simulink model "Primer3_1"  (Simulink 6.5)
settings: Solver=ode23t  SolverMode=SingleTasking  StartTime=0.0  StopTime=0.1  RelTol=1e-3  AbsTol=1e-6
undefined symbols (not defined in the file or in its folder): blocks, Continuous, powergui, ZData
libraries: powerlib x17

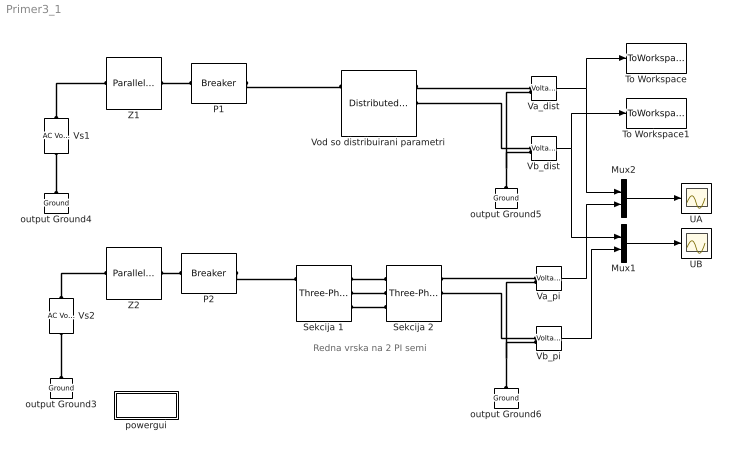
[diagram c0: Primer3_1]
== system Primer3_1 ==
  note: Redna vrska na 2 PI semi
  Mux1 : Mux  Inputs=2
  Mux2 : Mux  Inputs=2
  P1 : powerlib/Elements/Breaker  DialogController=PMDialogs.PMDefaultMaskDlg  SystemSampleTime=-1  BreakerResistance=0.01  InitialState=0  SnubberResistance=inf  SnubberCapacitance=inf  SwitchingTimes="[ 0.25/50  4/50 ]"  External=off  Measurements=None  MoreParameters=off  NoBreakLoop=off
  P2 : powerlib/Elements/Breaker  DialogController=PMDialogs.PMDefaultMaskDlg  SystemSampleTime=-1  BreakerResistance=0.01  InitialState=0  SnubberResistance=inf  SnubberCapacitance=inf  SwitchingTimes="[ 0.25/50  4/50 ]"  External=off  Measurements=None  MoreParameters=off  NoBreakLoop=off
  Sekcija 1 : powerlib/Elements/Three-Phase PI Section Line  DialogController=PMDialogs.PMDefaultMaskDlg  PhysicalDomain=powersysdomain  SubClassName=unknown  LeftPortType=p1  RightPortType=p1  LConnTagsString=a|b|c  RConnTagsString=A|B|C  Frequency=50  Resistances=[0.029983 0.29405]  Inductances=[0.0010055 0.0025377]  Capacitances=[1.1784e-008 8.6541e-009]  Length=113.5/2
  Sekcija 2 : powerlib/Elements/Three-Phase PI Section Line  DialogController=PMDialogs.PMDefaultMaskDlg  PhysicalDomain=powersysdomain  SubClassName=unknown  LeftPortType=p1  RightPortType=p1  LConnTagsString=a|b|c  RConnTagsString=A|B|C  Frequency=50  Resistances=[0.029983 0.29405]  Inductances=[0.0010055 0.0025377]  Capacitances=[1.1784e-008 8.6541e-009]  Length=113.5/2
  To Workspace : ToWorkspace  VariableName=ua  SampleTime=-1  SaveFormat=Array
  To Workspace1 : ToWorkspace  VariableName=ub  SampleTime=-1  SaveFormat=Array
  UA : Scope
  UB : Scope
  Va_dist : powerlib/Measurements/Voltage Measurement  Tag=PoWeRsYsTeMmEaSuReMeNt  DialogController=PMDialogs.PMDefaultMaskDlg  SystemSampleTime=-1  PhasorSimulation=off  OutputType=Magnitude  PSBequivalent=0
  Va_pi : powerlib/Measurements/Voltage Measurement  Tag=PoWeRsYsTeMmEaSuReMeNt  DialogController=PMDialogs.PMDefaultMaskDlg  SystemSampleTime=-1  PhasorSimulation=off  OutputType=Magnitude  PSBequivalent=0
  Vb_dist : powerlib/Measurements/Voltage Measurement  Tag=PoWeRsYsTeMmEaSuReMeNt  DialogController=PMDialogs.PMDefaultMaskDlg  SystemSampleTime=-1  PhasorSimulation=off  OutputType=Magnitude  PSBequivalent=0
  Vb_pi : powerlib/Measurements/Voltage Measurement  Tag=PoWeRsYsTeMmEaSuReMeNt  DialogController=PMDialogs.PMDefaultMaskDlg  SystemSampleTime=-1  PhasorSimulation=off  OutputType=Magnitude  PSBequivalent=0
  Vod so distribuirani parametri : powerlib/Elements/Distributed Parameters Line  DialogController=PMDialogs.PMDefaultMaskDlg  SystemSampleTime=-1  Phases=3  Frequency=50  Resistance=[0.029983 0.29405]  Inductance=[0.0010055 0.0025377]  Capacitance=[1.1784e-008 8.6541e-009]  Length=113.5  x1=[0 0 0 0;0.000106379256748321 0 0 0;0.000212758513496643 0 0 0;0.000319137770244964 0 0 0;0.000425517026993286 0 0 0;0.000531896283741607 0 0 0]  x2=[0 0 0 0;0.000106379256748321 0 0 0;0.000212758513496643 0 0 0;0.000319137770244964 0 0 0;0.000425517026993286 0 0 0;0.000531896283741607 0 0 0]  x3=[0 0 0 0;0.000106379256748321 0 0 0;0.000212758513496643 0 0 0;0.000319137770244964 0 0 0;0.000425517026993286 0 0 0;0.000531896283741607 0 0 0]  x4=[0 0 0 0;0.000106379256748321 0 0 0;0.000212758513496643 0 0 0;0.000319137770244964 0 0 0;0.000425517026993286 0 0 0;0.000531896283741607 0 0 0]  x5=0.000531896283741607  Measurements=None
  Vs1 : powerlib/Electrical Sources/AC Voltage Source  Description=source block  Orientation=up  DialogController=PMDialogs.PMDefaultMaskDlg  SystemSampleTime=-1  Amplitude=400e3/sqrt(3)*sqrt(2)  Phase=0  Frequency=50  SampleTime=0  Measurements=None
  Vs2 : powerlib/Electrical Sources/AC Voltage Source  Description=source block  Orientation=up  DialogController=PMDialogs.PMDefaultMaskDlg  SystemSampleTime=-1  Amplitude=400e3/sqrt(3)*sqrt(2)  Phase=0  Frequency=50  SampleTime=0  Measurements=None
  Z1 : powerlib/Elements/Parallel RLC Branch  DialogController=PMDialogs.PMDefaultMaskDlg  PhysicalDomain=powersysdomain  SubClassName=unknown  LeftPortType=p1  RightPortType=p1  LConnTagsString=a  RConnTagsString=__new0  BranchType=RL  Resistance=145.8  Inductance=46.4e-3  SetiL0=on  InitialCurrent=0  Capacitance=1e-6  Setx0=off  InitialVoltage=0  Measurements=None
  Z2 : powerlib/Elements/Parallel RLC Branch  DialogController=PMDialogs.PMDefaultMaskDlg  PhysicalDomain=powersysdomain  SubClassName=unknown  LeftPortType=p1  RightPortType=p1  LConnTagsString=a  RConnTagsString=__new0  BranchType=RL  Resistance=145.8  Inductance=46.4e-3  SetiL0=on  InitialCurrent=0  Capacitance=1e-6  Setx0=off  InitialVoltage=0  Measurements=None
  output Ground{3..6} (4 alike) : powerlib/Elements/Ground  Orientation=down  DialogController=PMDialogs.PMDefaultMaskDlg  PhysicalDomain=powersysdomain  SubClassName=unknown  LeftPortType=p1  RightPortType=p1  LConnTagsString=a
  powergui : Subsystem  AncestorBlock=powerlib/powergui  InitFcn=powergui( 'InitFcn_Callback' , gcb , 0 , [ ] );  mask(PSB option menu block){SimulationMode=Continuous, SampleTime=0, echomessages=off, RestoreLinks=warning, x0status=blocks, Frange=[0:2:500], Ylog=off, Xlog=on, ShowGrid=off, save=off, variable=ZData, structure=, ZoomFFT=on, StartTime=0.0, cycles=1, DisplayStyle=1, fundamental=60, FreqAxis=off, MaxFrequency=1000, frequencyindice=50, frequencyindicesteady=1, RmsSteady=1, display=off, Ts=0, frequency=60, methode=off, HookPort=off, Interpol=off}
      mask prompts: SimulationMode "Simulation mode"; SampleTime "Sample time Ts (when simulation mode is Discrete) (s)"; echomessages "Echo  Messages"; RestoreLinks "Restore disabled links"; x0status "Initial electrical states status"; Frange "Impedance tool: Frequency Range"; Ylog "Impedance tool: Log impedance"; Xlog "Impedance tool: log Frequency"; ShowGrid "Impedance tool: grid"; save "Impedance tool: Save Data To Workspace"; variable "Impedance tool: Variable Name"; structure "Structure Name (PSBFFTSCOPE)"; ZoomFFT "ZoomFFT (PSBFFTSCOPE)"; StartTime "Start Time (PSBFFTSCOPE)"; cycles "Cycles (PSBFFTSCOPE)"; DisplayStyle "Display style (PSBFFTSCOPE)"; fundamental "Fundamental (PSBFFTSCOPE)"; FreqAxis "Frequency Axis (PSBFFTSCOPE)"; MaxFrequency "Max Frequency (PSBFFTSCOPE)"; frequencyindice "Load flow frequency (Hz)"; frequencyindicesteady "Frequency indice (STEADYSTATE)"; RmsSteady "RMS display (STEADYSTATE)"; display "Display Results"; Ts "OBSOLETE 1"; frequency "Phasor frequency (Hz)"; methode "Phasor simulation"; HookPort "Hook port"; Interpol "Interpolate"
      mask init:
      | powerlibroot = which('powersysdomain');
      | PSBroot = powerlibroot(1:end-16);
      | %
      | switch SimulationMode
      | 	case 1
      | 		message=sprintf('Continuous');
      | 	case 2
      |         SampleTimeeval=evalin('base',SampleTime,'NaN');
      |         if isnan(SampleTimeeval)
      |             message=sprintf('Warning !!,\nUndefined sample time');
      |         else
      |             message=sprintf('Discrete,\nTs = %.4g s.',SampleTimeeval);
      |         end
      | 	case 3
      | 		message=sprintf('Phasors');
      | end
      | if strcmp(bdroot,'powerlib')
      |   message='powergui';
      | end
      | power_initmask();
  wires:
  Vb_dist/1 -> Mux1/1, To Workspace1/1
  Va_dist/1 -> Mux2/1, To Workspace/1
  Vb_pi/1 -> Mux1/2
  Va_pi/1 -> Mux2/2
  Mux2/1 -> UA/1
  Mux1/1 -> UB/1
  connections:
  Vod so distribuirani parametri/RConn1 -- Va_dist/LConn1
  Vod so distribuirani parametri/RConn2 -- Vb_dist/LConn1
  output Ground5/LConn1 -- Vb_dist/LConn2 -- Va_dist/LConn2
  P1/RConn1 -- Vod so distribuirani parametri/LConn1
  output Ground6/LConn1 -- Va_pi/LConn2 -- Vb_pi/LConn2
  Sekcija 2/RConn2 -- Vb_pi/LConn1
  Sekcija 2/RConn1 -- Va_pi/LConn1
  Sekcija 1/RConn3 -- Sekcija 2/LConn3
  Sekcija 1/RConn2 -- Sekcija 2/LConn2
  Sekcija 1/RConn1 -- Sekcija 2/LConn1
  P2/RConn1 -- Sekcija 1/LConn1
  Z2/RConn1 -- P2/LConn1
  Z1/RConn1 -- P1/LConn1
  output Ground4/LConn1 -- Vs1/LConn1
  output Ground3/LConn1 -- Vs2/LConn1
  Vs1/RConn1 -- Z1/LConn1
  Vs2/RConn1 -- Z2/LConn1

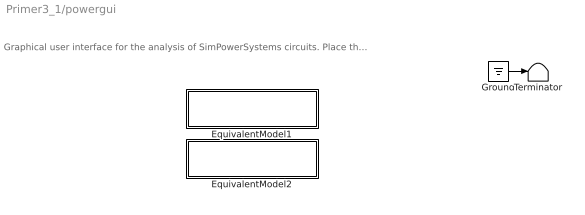
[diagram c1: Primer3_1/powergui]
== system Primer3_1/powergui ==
  note: Graphical user interface for the analysis of SimPowerSystems circuits. Place the Powergui block in the top-level of your model and double-click on it to open the GUI.
  EquivalentModel1 : Subsystem
  EquivalentModel2 : Subsystem
  Ground : Ground
  Terminator : Terminator
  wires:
  Ground/1 -> Terminator/1

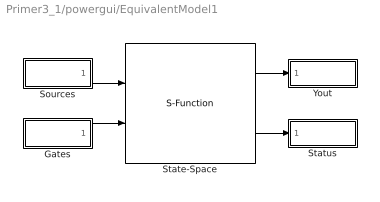
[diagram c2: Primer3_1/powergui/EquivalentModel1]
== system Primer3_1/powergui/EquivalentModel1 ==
  Gates : Subsystem
  Sources : Subsystem
  State-Space : S-Function  FunctionName=sfun_spssw_contc  Parameters=A, B, C, D, x0, SwitchResistance ,SwitchType, SwitchGateInitialValue, OutputsToResetToZero
  Status : Subsystem
  Yout : Subsystem
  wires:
  Gates/1(gates) -> State-Space/2
  Sources/1(u) -> State-Space/1
  State-Space/2 -> Status/1(status)
  State-Space/1 -> Yout/1(v,i)

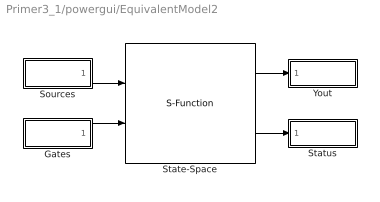
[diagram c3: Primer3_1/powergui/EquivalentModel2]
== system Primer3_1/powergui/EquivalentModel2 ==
  Gates : Subsystem
  Sources : Subsystem
  State-Space : S-Function  FunctionName=sfun_spssw_contc  Parameters=A, B, C, D, x0, SwitchResistance ,SwitchType, SwitchGateInitialValue, OutputsToResetToZero
  Status : Subsystem
  Yout : Subsystem
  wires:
  Gates/1(gates) -> State-Space/2
  Sources/1(u) -> State-Space/1
  State-Space/2 -> Status/1(status)
  State-Space/1 -> Yout/1(v,i)

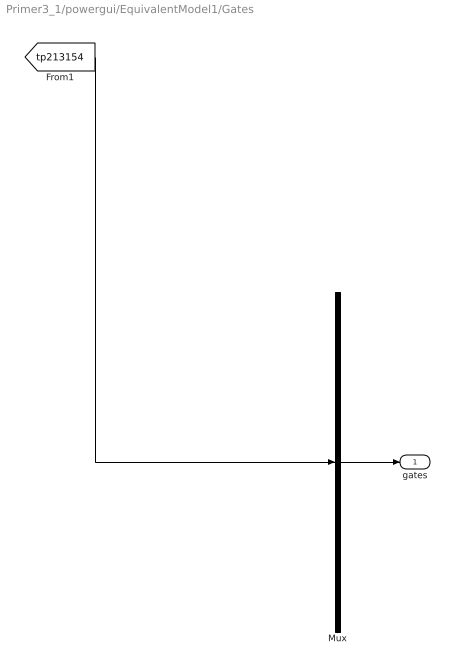
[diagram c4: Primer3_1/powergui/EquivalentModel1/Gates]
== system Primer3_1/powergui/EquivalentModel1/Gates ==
  Mux : Mux  Inputs=1
  gates : Outport
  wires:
  Mux/1 -> gates/1
  [tp213154] -> Mux/1

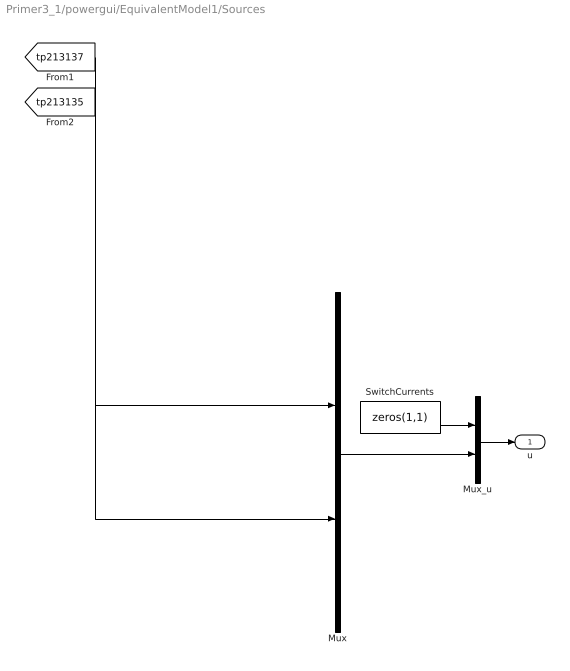
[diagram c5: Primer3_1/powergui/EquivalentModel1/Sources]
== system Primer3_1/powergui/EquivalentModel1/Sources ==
  Mux : Mux  Inputs=[6 1]
  Mux_u : Mux  Inputs=[1 7]
  SwitchCurrents : Constant  Value=zeros(1,1)  OutDataType=sfix(16)  ConRadixGroup=Use specified scaling  OutScaling=2^0  SampleTime=inf  FramePeriod=inf
  u : Outport
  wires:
  Mux/1 -> Mux_u/2
  SwitchCurrents/1 -> Mux_u/1
  Mux_u/1 -> u/1
  [tp213137] -> Mux/1
  [tp213135] -> Mux/2

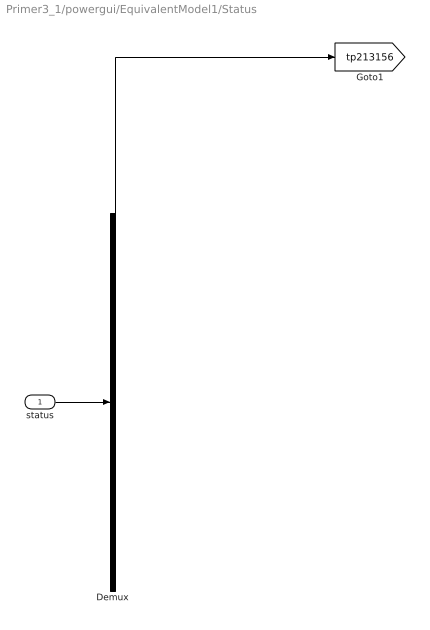
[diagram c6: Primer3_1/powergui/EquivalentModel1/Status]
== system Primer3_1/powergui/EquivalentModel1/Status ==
  status : Inport
  Demux : Demux  Outputs=1
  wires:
  status/1 -> Demux/1
  Demux/1 -> [tp213156]

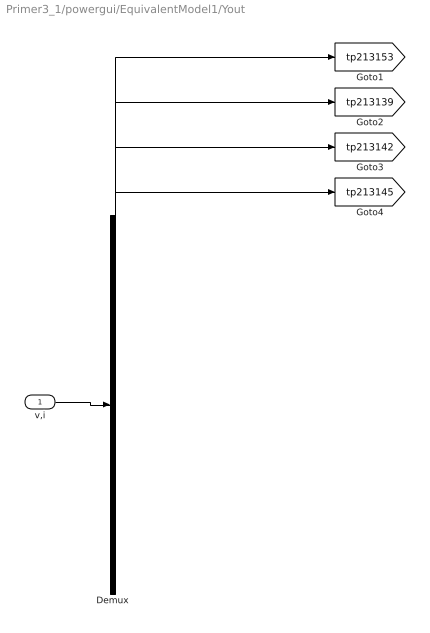
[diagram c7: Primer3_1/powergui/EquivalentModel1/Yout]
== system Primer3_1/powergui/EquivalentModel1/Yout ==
  v,i : Inport
  Demux : Demux  Outputs=[1 6 1 1]
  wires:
  v,i/1 -> Demux/1
  Demux/1 -> [tp213153]
  Demux/2 -> [tp213139]
  Demux/3 -> [tp213142]
  Demux/4 -> [tp213145]

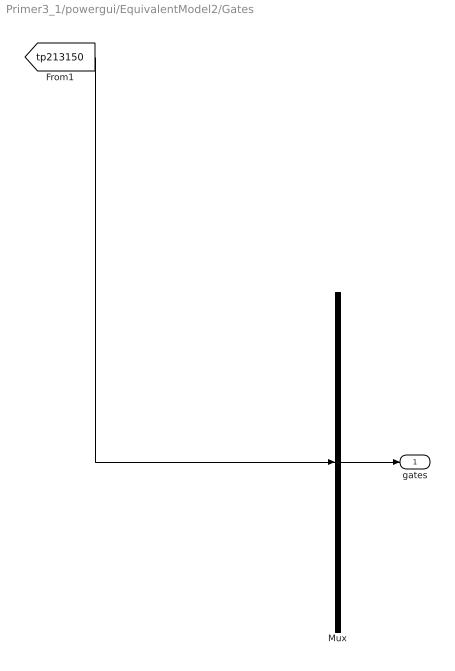
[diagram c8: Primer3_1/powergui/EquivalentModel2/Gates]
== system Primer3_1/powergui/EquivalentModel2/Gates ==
  Mux : Mux  Inputs=1
  gates : Outport
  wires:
  Mux/1 -> gates/1
  [tp213150] -> Mux/1

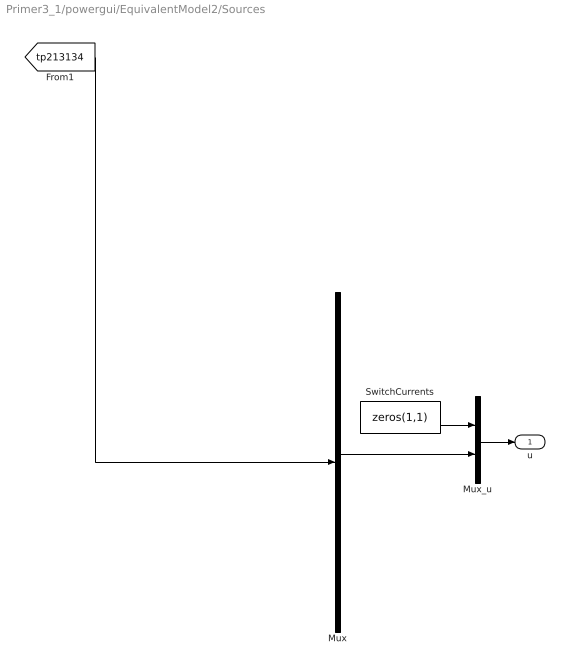
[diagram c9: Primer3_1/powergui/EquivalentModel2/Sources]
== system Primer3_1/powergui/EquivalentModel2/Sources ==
  Mux : Mux  Inputs=1
  Mux_u : Mux  Inputs=[1 1]
  SwitchCurrents : Constant  Value=zeros(1,1)  OutDataType=sfix(16)  ConRadixGroup=Use specified scaling  OutScaling=2^0  SampleTime=inf  FramePeriod=inf
  u : Outport
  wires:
  Mux/1 -> Mux_u/2
  SwitchCurrents/1 -> Mux_u/1
  Mux_u/1 -> u/1
  [tp213134] -> Mux/1

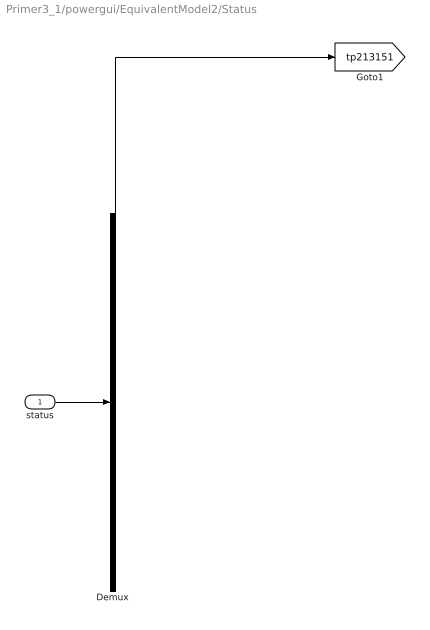
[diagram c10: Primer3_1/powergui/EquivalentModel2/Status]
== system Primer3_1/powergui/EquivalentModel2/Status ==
  status : Inport
  Demux : Demux  Outputs=1
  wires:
  status/1 -> Demux/1
  Demux/1 -> [tp213151]

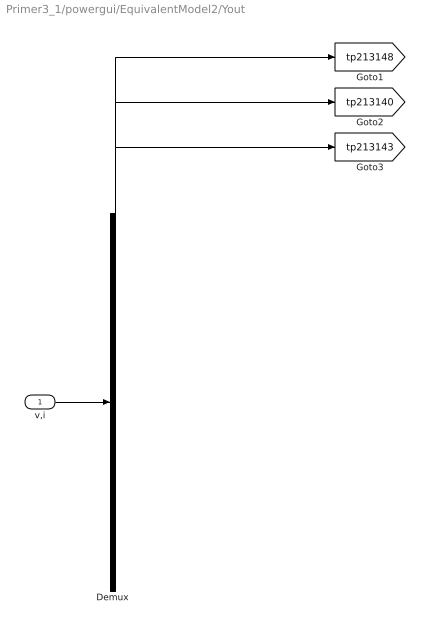
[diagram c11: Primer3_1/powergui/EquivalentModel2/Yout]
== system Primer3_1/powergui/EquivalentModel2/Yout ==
  v,i : Inport
  Demux : Demux  Outputs=[1 1 1]
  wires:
  v,i/1 -> Demux/1
  Demux/1 -> [tp213148]
  Demux/2 -> [tp213140]
  Demux/3 -> [tp213143]
